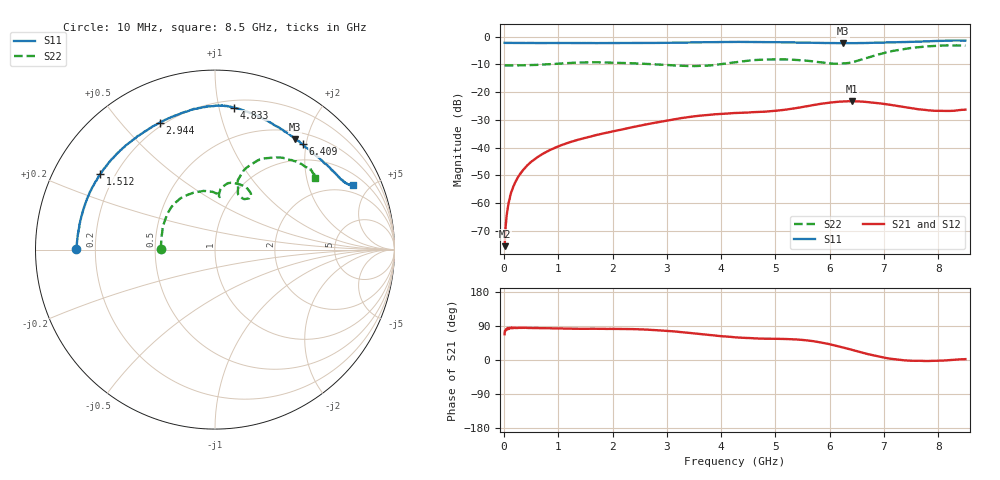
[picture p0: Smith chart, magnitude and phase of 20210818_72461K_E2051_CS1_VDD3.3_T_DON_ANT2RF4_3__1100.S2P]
!Agilent Technologies,E5071C,MY46417908,A.11.23
!Date: Wed Aug 18 14:33:05 2021
!Data & Calibration Information:
!Freq	S11:SOLT2(ON)	S21:SOLT2(ON)	S12:SOLT2(ON)	S22:SOLT2(ON)
!PortZ  Port1:50+j0  Port2:50+j0
!Above PortZ is port z conversion or system Z0 setting when saving the data.
!When reading, reference impedance value at option line is always used.
# Hz S dB R 50
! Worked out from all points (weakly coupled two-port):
!   1601 points, 10 MHz to 8.5 GHz, reference 50 ohm
!   highest |S21| = -23.30 dB at 6.409 GHz (marker M1); lowest = -75.6 dB at 10 MHz (marker M2)
!   lowest |S11| = -2.4 dB at 6.25 GHz (marker M3), VSWR 7.33, Z = 30.8 + j89.8 ohm
!   |S11| at or under -10 dB: nowhere
!   |S22| runs from -10.6 to -3.1 dB; largest |S21 - S12| = 0.00034
!   S11 on the Smith chart (normalised r, x): 10 MHz: 0.13, +0.00; 1.512 GHz: 0.14, +0.29; 2.944 GHz: 0.18, +0.64; 4.833 GHz: 0.26, +1.11; 6.409 GHz: 0.69, +1.94; 8.5 GHz: 1.52, +3.93
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1e7  -2.23 179.7  -75.56 67.9  -76.71 73.9  -10.36 179.5
6.836875e7  -2.26 178.4  -61.74 84.4  -61.54 82.5  -10.38 177.8
1.214312e8  -2.27 177.1  -57.03 84.2  -56.81 84.2  -10.39 176.1
2.116375e8  -2.29 175.0  -52.30 84.6  -52.28 84.6  -10.39 173.5
3.389875e8  -2.29 172.2  -48.39 84.6  -48.37 85.1  -10.34 170.1
5.087875e8  -2.31 168.4  -44.98 84.3  -45.01 84.4  -10.26 165.6
7.581812e8  -2.31 162.8  -41.79 83.9  -41.80 84.1  -10.01 157.4
1.426769e9  -2.32 148.5  -36.87 82.2  -36.87 82.4  -9.33 132.4
1.511669e9  -2.32 146.6  -36.42 82.5  -36.45 82.4  -9.31 129.1
2.843538e9  -2.27 115.8  -30.84 78.5  -30.84 78.4  -10.08 88.6
2.944356e9  -2.26 113.5  -30.46 77.6  -30.45 77.6  -10.15 87.3
3.53335e9  -2.09 101.3  -28.66 69.6  -28.66 69.7  -10.60 85.1
4.255e9  -1.93 89.9  -27.56 60.0  -27.56 59.9  -9.28 84.3
4.833381e9  -1.96 82.3  -27.02 56.2  -27.02 56.2  -8.26 73.7
5.671769e9  -2.22 67.6  -24.78 50.3  -24.79 50.4  -8.88 56.5
6.25015e9  -2.38 54.0  -23.41 32.9  -23.43 32.9  -9.68 65.0
6.409338e9  -2.33 50.2  -23.30 26.7  -23.32 26.7  -9.26 68.2
6.706488e9  -2.29 42.8  -23.61 15.4  -23.64 15.4  -7.57 71.5
7.088538e9  -2.09 35.5  -24.51 4.0  -24.55 3.8  -5.50 65.7
7.534262e9  -1.87 28.9  -25.93 -2.1  -25.93 -2.1  -4.02 54.6
8.022438e9  -1.53 25.5  -26.76 -1.8  -26.75 -1.9  -3.27 41.9
8.5e9  -1.42 25.1  -26.33 2.3  -26.35 2.0  -3.28 35.8
